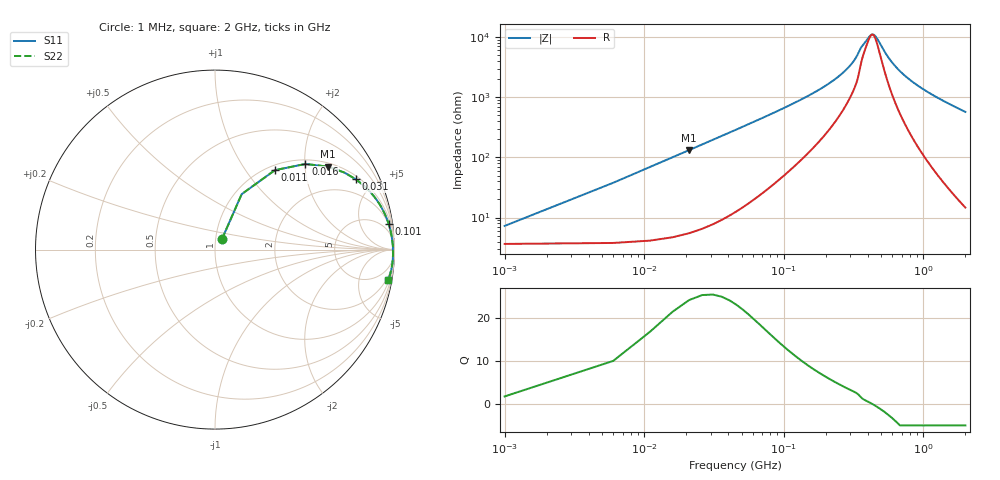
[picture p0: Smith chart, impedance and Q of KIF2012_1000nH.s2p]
!version-2
!date-12.2020
!Series
# MHz S RI R 50
!Freq ReS11 ImS11 ReS21 ImS21 ReS12 ImS12 ReS22 ImS22
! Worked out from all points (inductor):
!   401 points, 1 MHz to 2 GHz, reference 50 ohm
!   read as one part in series: L = 1 uH near 11 MHz
!   highest Q = 23.9 at 21 MHz (marker M1), where L = 1 uH
!   self-resonance near 426 MHz
!   S11 on the Smith chart (normalised r, x): 1 MHz: 1.07, +0.13; 11 MHz: 1.08, +1.38; 16 MHz: 1.09, +2.01; 31 MHz: 1.15, +3.91; 101 MHz: 2, +13; 2 GHz: 1, -11
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1  0.0387 0.0582  0.9613 -0.0582  0.9613 -0.0582  0.0387 0.0582
11  0.3335 0.4425  0.6665 -0.4425  0.6665 -0.4425  0.3335 0.4425
16  0.5035 0.4771  0.4965 -0.4771  0.4965 -0.4771  0.5035 0.4771
21  0.6312 0.4621  0.3688 -0.4621  0.3688 -0.4621  0.6312 0.4621
31  0.784 0.3922  0.216 -0.3922  0.216 -0.3922  0.784 0.3922
41  0.8609 0.3258  0.1391 -0.3258  0.1391 -0.3258  0.8609 0.3258
56  0.917 0.2528  0.083 -0.2528  0.083 -0.2528  0.917 0.2528
101  0.9677 0.1428  0.0323 -0.1428  0.0323 -0.1428  0.9677 0.1428
156  0.9819 0.0867  0.0181 -0.0867  0.0181 -0.0867  0.9819 0.0867
291  0.9903 0.03  0.00974 -0.03  0.00974 -0.03  0.9903 0.03
336  0.992 0.0182  0.00802 -0.0182  0.00802 -0.0182  0.992 0.0182
361  0.9914 0.0115  0.00858 -0.0115  0.00858 -0.0115  0.9914 0.0115
401  0.9907 0.00473  0.00926 -0.00473  0.00926 -0.00473  0.9907 0.00473
436  0.9911 -0.00107  0.00892 0.00107  0.00892 0.00107  0.9911 -0.00107
461  0.9913 -0.0051  0.0087 0.0051  0.0087 0.0051  0.9913 -0.0051
566  0.9917 -0.0206  0.00828 0.0206  0.00828 0.0206  0.9917 -0.0206
671  0.9916 -0.0345  0.0084 0.0345  0.0084 0.0345  0.9916 -0.0345
811  0.9908 -0.0513  0.00918 0.0513  0.00918 0.0513  0.9908 -0.0513
1001  0.9888 -0.0724  0.0112 0.0724  0.0112 0.0724  0.9888 -0.0724
1336  0.9833 -0.1067  0.0167 0.1067  0.0167 0.1067  0.9833 -0.1067
1671  0.9756 -0.1387  0.0244 0.1387  0.0244 0.1387  0.9756 -0.1387
2000  0.9661 -0.1685  0.0339 0.1685  0.0339 0.1685  0.9661 -0.1685
